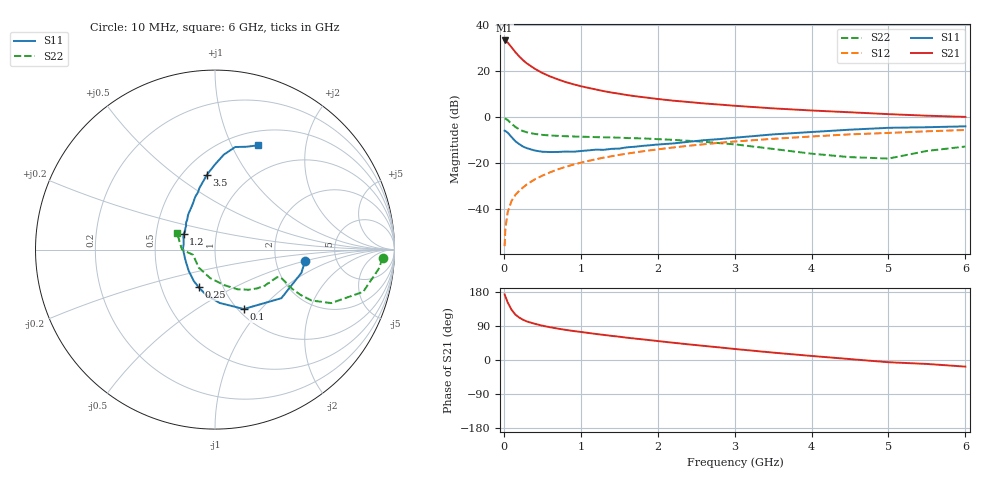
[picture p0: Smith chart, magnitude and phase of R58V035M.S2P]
! SIEMENS Small Signal Semiconductors
! BFR183
! Si NPN RF Bipolar Junction Transistor in SOT23
! VCE = 8 V  IC = 35 mA
! Common Emitter S-Parameters:  May  1996
# GHz  S  MA  R  50
!  f  S11  S21  S12  S22
! GHz  MAG  ANG  MAG  ANG  MAG  ANG  MAG  ANG
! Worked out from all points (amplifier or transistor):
!   36 points, 10 MHz to 6 GHz, reference 50 ohm
!   highest |S21| = 33.1 dB at 10 MHz (marker M1)
!   |S21| within 3 dB of that: start of sweep to 101.2 MHz
!   unconditionally stable (mu >= 1): 473.2 MHz to 2.449 GHz
!   at 250 MHz: K = 0.88, MSG = 27.5 dB, |S12| = -30.5 dB
!   at 1.4 GHz: K = 1.04, MAG = 12.5 dB, |S12| = -17.0 dB
!   at 6 GHz: K = 0.90, MSG = 2.8 dB, |S12| = -5.6 dB
!   S11 on the Smith chart (normalised r, x): 10 MHz: 2.96, -0.50; 100 MHz: 1.06, -0.81; 250 MHz: 0.77, -0.34; 1.2 GHz: 0.69, +0.13; 3.5 GHz: 0.65, +0.66; 6 GHz: 0.66, +1.26
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0.01  0.5063 -7.1  45.26 173.2  0.0016 82.4  0.9348 -2.9
0.02  0.4984 -15.1  44.6 167.5  0.0038 82.2  0.9184 -6.7
0.05  0.4584 -36.2  40.85 152.1  0.0088 76.5  0.8585 -15.9
0.1  0.3679 -64.2  32.23 132.8  0.0152 71.7  0.713 -24.7
0.15  0.2984 -85.0  25.25 119.8  0.0206 69.3  0.6085 -27.8
0.2  0.2586 -100.6  20.41 111.9  0.0252 70.8  0.5394 -27.9
0.25  0.2288 -113.4  16.89 106.1  0.0299 70.7  0.4935 -27.2
0.3  0.211 -124.1  14.42 101.7  0.0348 72.3  0.4658 -26.4
0.4  0.1882 -141.1  11.11 95.7  0.0444 73.3  0.4302 -24.6
0.5  0.1767 -155.0  8.96 90.6  0.0536 73.5  0.4094 -23.6
0.6  0.1743 -163.8  7.549 86.5  0.0633 73.6  0.3982 -23.2
0.7  0.1748 -173.9  6.53 82.9  0.0733 73.2  0.3903 -23.4
0.8  0.1785 177.7  5.725 79.6  0.0829 72.6  0.3835 -23.7
0.9  0.1769 170.9  5.12 76.6  0.0928 72.1  0.3781 -24.0
1.1  0.1894 158.3  4.256 71.4  0.112 70.3  0.3701 -26.3
1.2  0.1961 153.4  3.924 68.6  0.122 69.5  0.3662 -27.2
1.6  0.2203 137.0  2.983 58.8  0.1608 65.4  0.35 -32.5
2.2  0.2673 119.9  2.254 45.6  0.2184 58.7  0.3203 -42.4
3.5  0.4198 96.1  1.535 19.5  0.3364 42.2  0.2035 -75.9
4.5  0.5311 84.7  1.263 2.4  0.4205 29.6  0.1352 -132.0
5.5  0.5996 72.9  1.065 -10.4  0.4896 18.2  0.1841 -179.8
6  0.6271 67.8  1.004 -17.5  0.5226 10.8  0.2291 156.8
